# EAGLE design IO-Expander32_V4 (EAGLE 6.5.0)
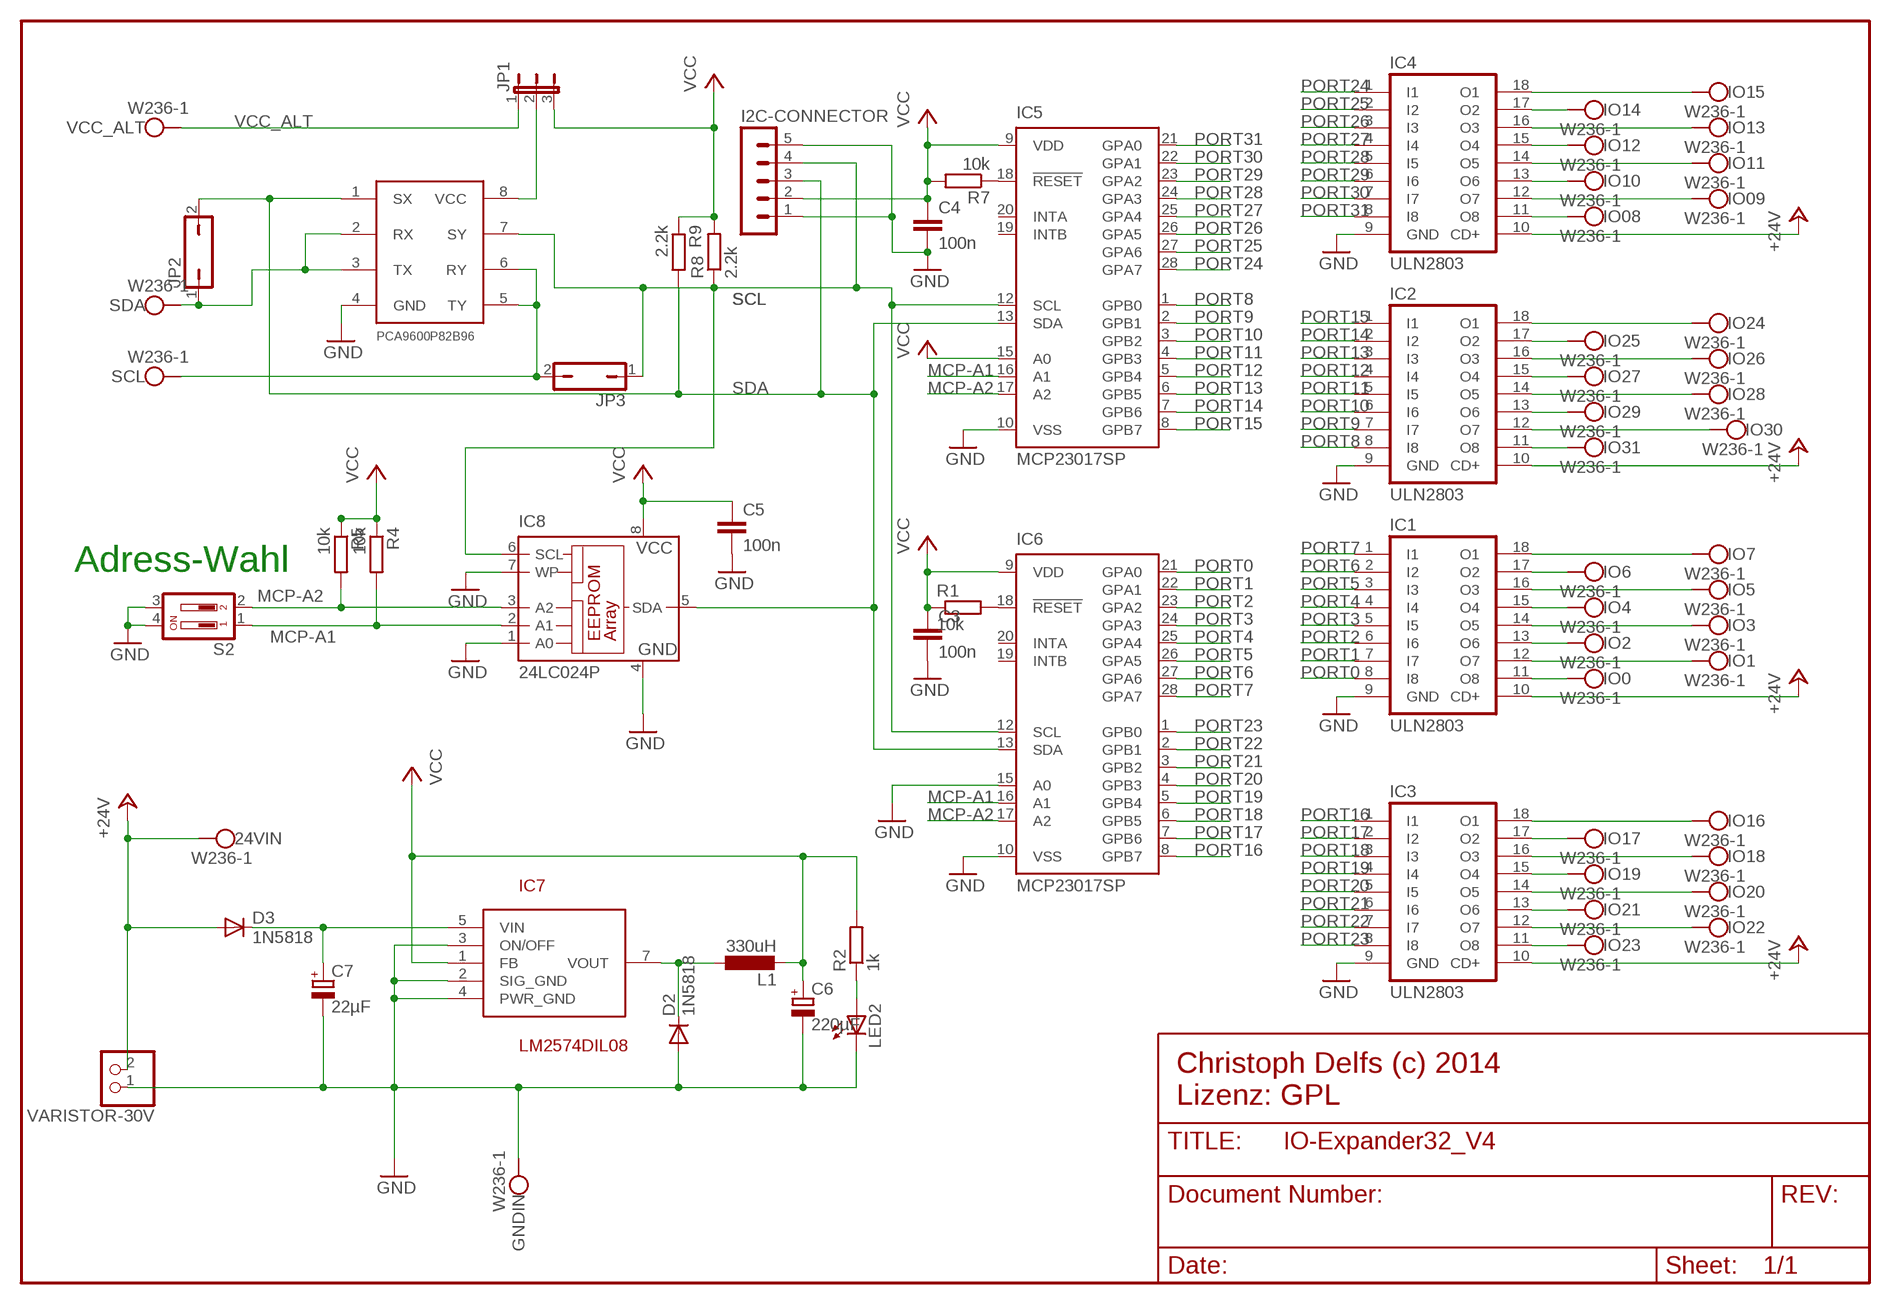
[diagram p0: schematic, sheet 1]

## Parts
24VIN  W236-1  [W236-1]
C3  100n  C-EU050-025X075  [C050-025X075]
C4  100n  C-EU050-025X075  [C050-025X075]
C5  100n  C-EU050-025X075  [C050-025X075]
C6  220µF  CPOL-EUE5-10.5  [E5-10,5]
C7  22µF  CPOL-EUE2.5-6  [E2,5-6]
D2  1N5818  1N4148  [DO35-10]
D3  1N5818  1N4148  [DO35-10]
GNDIN  W236-1  [W236-1]
I2C-CONNECTOR  MA05-1  [MA05-1]
IC1  ULN2803  ULN2803A  [DIL18]
IC2  ULN2803  ULN2803A  [DIL18]
IC3  ULN2803  ULN2803A  [DIL18]
IC4  ULN2803  ULN2803A  [DIL18]
IC5  MCP23017SP  [DIL28-3]
IC6  MCP23017SP  [DIL28-3]
IC7  LM2574DIL08  [DIL08]
IC8  24LC024P  [DIL8]
IO0  W236-1  [W236-1]
IO1  W236-1  [W236-1]
IO2  W236-1  [W236-1]
IO3  W236-1  [W236-1]
IO4  W236-1  [W236-1]
IO5  W236-1  [W236-1]
IO6  W236-1  [W236-1]
IO7  W236-1  [W236-1]
IO08  W236-1  [W236-1]
IO09  W236-1  [W236-1]
IO10  W236-1  [W236-1]
IO11  W236-1  [W236-1]
IO12  W236-1  [W236-1]
IO13  W236-1  [W236-1]
IO14  W236-1  [W236-1]
IO15  W236-1  [W236-1]
IO16  W236-1  [W236-1]
IO17  W236-1  [W236-1]
IO18  W236-1  [W236-1]
IO19  W236-1  [W236-1]
IO20  W236-1  [W236-1]
IO21  W236-1  [W236-1]
IO22  W236-1  [W236-1]
IO23  W236-1  [W236-1]
IO24  W236-1  [W236-1]
IO25  W236-1  [W236-1]
IO26  W236-1  [W236-1]
IO27  W236-1  [W236-1]
IO28  W236-1  [W236-1]
IO29  W236-1  [W236-1]
IO30  W236-1  [W236-1]
IO31  W236-1  [W236-1]
JP1  JP2E  [JP2]
JP2  JP1Q  [JP1]
JP3  JP1Q  [JP1]
L1  330uH  L-EU2200-12.7  [2200-12.7]
LED2  LED3MM  [LED3MM]
PCA9600  PCA9600  P82B96  [SOIC8]
R1  10k  R-EU_0207/2V  [0207/2V]
R2  1k  R-EU_0207/10  [0207/10]
R4  10k  R-EU_0207/7  [0207/7]
R5  10k  R-EU_0207/7  [0207/7]
R7  10k  R-EU_0207/7  [0207/7]
R8  2.2k  R-EU_0207/7  [0207/7]
R9  2.2k  R-EU_0207/7  [0207/7]
S2  DIP02YL  [DIP02YL]
SCL  W236-1  [W236-1]
SDA  W236-1  [W236-1]
VARISTOR-30V  PINHD-1X2  [1X02]
VCC_ALT  W236-1  [W236-1]

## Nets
+24V: 24VIN.1(KL1) D3.A IC1.10(CD+) IC2.10(CD+) IC3.10(CD+) IC4.10(CD+) VARISTOR-30V.2
GND: C3.2 C4.2 C5.2 C6.- C7.- D2.A GNDIN.1(KL1) I2C-CONNECTOR.1 I2C-CONNECTOR.5 IC1.9(GND) IC2.9(GND) IC3.9(GND) IC4.9(GND) IC5.10(VSS) IC6.10(VSS) IC6.15(A0) IC7.2(SIG_GND) IC7.3(ON/OFF) IC7.4(PWR_GND) IC8.1(A0) IC8.4(GND) IC8.7(WP) LED2.K(C) PCA9600.4(GND) S2.3 S2.4 VARISTOR-30V.1
IO1: IC1.18(O1) IO7.1(KL1)
IO2: IC3.16(O3) IO18.1(KL1)
IO14: IC2.16(O3) IO26.1(KL1)
IO24: IC4.18(O1) IO15.1(KL1)
MCP-A1: IC5.16(A1) IC6.16(A1) IC8.2(A1) R4.2 S2.1
MCP-A2: IC5.17(A2) IC6.17(A2) IC8.3(A2) R5.2 S2.2
N$1: LED2.A R2.1
N$2: IC6.18(!RESET) R1.2
N$4: IC4.17(O2) IO14.1(KL1)
N$5: IC4.16(O3) IO13.1(KL1)
N$7: IC4.15(O4) IO12.1(KL1)
N$8: IC4.14(O5) IO11.1(KL1)
N$9: IC4.13(O6) IO10.1(KL1)
N$10: IC4.12(O7) IO09.1(KL1)
N$11: IC5.18(!RESET) R7.1
N$12: JP1.2 PCA9600.8(VCC)
N$14: JP3.2 PCA9600.5(TY) PCA9600.6(RY) SCL.1(KL1)
N$16: JP2.1 PCA9600.2(RX) PCA9600.3(TX) SDA.1(KL1)
N$17: IC1.17(O2) IO6.1(KL1)
N$18: IC1.16(O3) IO5.1(KL1)
N$19: IC1.15(O4) IO4.1(KL1)
N$20: IC1.14(O5) IO3.1(KL1)
N$21: IC1.13(O6) IO2.1(KL1)
N$22: IC1.12(O7) IO1.1(KL1)
N$23: IC1.11(O8) IO0.1(KL1)
N$24: IC3.18(O1) IO16.1(KL1)
N$25: IC3.17(O2) IO17.1(KL1)
N$26: IC3.15(O4) IO19.1(KL1)
N$27: IC3.14(O5) IO20.1(KL1)
N$28: IC3.13(O6) IO21.1(KL1)
N$29: IC3.12(O7) IO22.1(KL1)
N$30: IC3.11(O8) IO23.1(KL1)
N$43: C7.+ D3.C IC7.5(VIN)
N$50: D2.C IC7.7(VOUT) L1.1
N$56: IC4.11(O8) IO08.1(KL1)
N$65: IC2.18(O1) IO24.1(KL1)
N$66: IC2.17(O2) IO25.1(KL1)
N$68: IC2.15(O4) IO27.1(KL1)
N$69: IC2.14(O5) IO28.1(KL1)
N$70: IC2.13(O6) IO29.1(KL1)
N$71: IC2.12(O7) IO30.1(KL1)
N$72: IC2.11(O8) IO31.1(KL1)
PORT0: IC1.8(I8) IC6.21(GPA0)
PORT1: IC1.7(I7) IC6.22(GPA1)
PORT2: IC1.6(I6) IC6.23(GPA2)
PORT3: IC1.5(I5) IC6.24(GPA3)
PORT4: IC1.4(I4) IC6.25(GPA4)
PORT5: IC1.3(I3) IC6.26(GPA5)
PORT6: IC1.2(I2) IC6.27(GPA6)
PORT7: IC1.1(I1) IC6.28(GPA7)
PORT8: IC2.8(I8) IC5.1(GPB0)
PORT9: IC2.7(I7) IC5.2(GPB1)
PORT10: IC2.6(I6) IC5.3(GPB2)
PORT11: IC2.5(I5) IC5.4(GPB3)
PORT12: IC2.4(I4) IC5.5(GPB4)
PORT13: IC2.3(I3) IC5.6(GPB5)
PORT14: IC2.2(I2) IC5.7(GPB6)
PORT15: IC2.1(I1) IC5.8(GPB7)
PORT16: IC3.1(I1) IC6.8(GPB7)
PORT17: IC3.2(I2) IC6.7(GPB6)
PORT18: IC3.3(I3) IC6.6(GPB5)
PORT19: IC3.4(I4) IC6.5(GPB4)
PORT20: IC3.5(I5) IC6.4(GPB3)
PORT21: IC3.6(I6) IC6.3(GPB2)
PORT22: IC3.7(I7) IC6.2(GPB1)
PORT23: IC3.8(I8) IC6.1(GPB0)
PORT24: IC4.1(I1) IC5.28(GPA7)
PORT25: IC4.2(I2) IC5.27(GPA6)
PORT26: IC4.3(I3) IC5.26(GPA5)
PORT27: IC4.4(I4) IC5.25(GPA4)
PORT28: IC4.5(I5) IC5.24(GPA3)
PORT29: IC4.6(I6) IC5.23(GPA2)
PORT30: IC4.7(I7) IC5.22(GPA1)
PORT31: IC4.8(I8) IC5.21(GPA0)
SCL: I2C-CONNECTOR.4 IC5.12(SCL) IC6.12(SCL) IC8.6(SCL) JP3.1 PCA9600.7(SY) R8.1
SDA: I2C-CONNECTOR.3 IC5.13(SDA) IC6.13(SDA) IC8.5(SDA) JP2.2 PCA9600.1(SX) R9.2
VCC: C3.1 C4.1 C5.1 C6.+ I2C-CONNECTOR.2 IC5.9(VDD) IC5.15(A0) IC6.9(VDD) IC7.1(FB) IC8.8(VCC) JP1.3 L1.2 R1.1 R2.2 R4.1 R5.1 R7.2 R8.2 R9.1
VCC_ALT: JP1.1 VCC_ALT.1(KL1)
Unconnected: 24VIN.2(KL2) GNDIN.2(KL2) IC5.19(INTB) IC5.20(INTA) IC6.19(INTB) IC6.20(INTA) IO0.2(KL2) IO1.2(KL2) IO2.2(KL2) IO3.2(KL2) IO4.2(KL2) IO5.2(KL2) IO6.2(KL2) IO7.2(KL2) IO08.2(KL2) IO09.2(KL2) IO10.2(KL2) IO11.2(KL2) IO12.2(KL2) IO13.2(KL2) IO14.2(KL2) IO15.2(KL2) IO16.2(KL2) IO17.2(KL2) IO18.2(KL2) IO19.2(KL2) IO20.2(KL2) IO21.2(KL2) IO22.2(KL2) IO23.2(KL2) IO24.2(KL2) IO25.2(KL2) IO26.2(KL2) IO27.2(KL2) IO28.2(KL2) IO29.2(KL2) IO30.2(KL2) IO31.2(KL2) SCL.2(KL2) SDA.2(KL2) VCC_ALT.2(KL2)

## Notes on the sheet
- Adress-Wahl
- Christoph Delfs (c) 2014
  Lizenz: GPL

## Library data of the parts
24VIN GNDIN IO0 IO1-IO7 IO08 IO09 IO10-IO31 SCL SDA VCC_ALT = con-wago-508:W236-1: WAGO SREW CLAMP
C3-C5 = rcl:C-EU: CAPACITOR, European symbol
C6 C7 = rcl:CPOL-EU: POLARIZED CAPACITOR, European symbol
D2 D3 = diode:1N4148: DIODE
I2C-CONNECTOR = con-lstb:MA05-1: PIN HEADER; OC_FARNELL: unknown; OC_NEWARK: unknown
IC1-IC4 = uln-udn:ULN2803A: DRIVER ARRAY
IC5 IC6 = microchip:MCP23017: http://ww1.microchip.com/downloads/en/DeviceDoc/21952a.pdf Source: http://ww1.microchip.com/downloads/en/DeviceDoc/21952a.pdf; MF: MICROCHIP; MPN: MCP23017-E/SP; OC_FARNELL: 1332088; OC_NEWARK: 31K2959
IC7 = hausbus-bauteile:LM2574
IC8 = microchip:24*: Serial EEPROM I2C; MPN: 24LC024-I/P; OC_FARNELL: 1331317; OC_NEWARK: 35M0731
JP1 = jumper:JP2E: JUMPER
JP2 JP3 = jumper:JP1Q: JUMPER
L1 = rcl:L-EU: INDUCTOR, European symbol
LED2 = led:LED: LED
PCA9600 = P82B96:P82B96: P82B96 - I2C buffer
R1 R2 R4 R5 R7-R9 = rcl:R-EU_: RESISTOR, European symbol
S2 = switch-dil:DIP02YL: DIL/CODE SWITCH; OC_FARNELL: unknown; OC_NEWARK: unknown
VARISTOR-30V = pinhead:PINHD-1X2: PIN HEADER

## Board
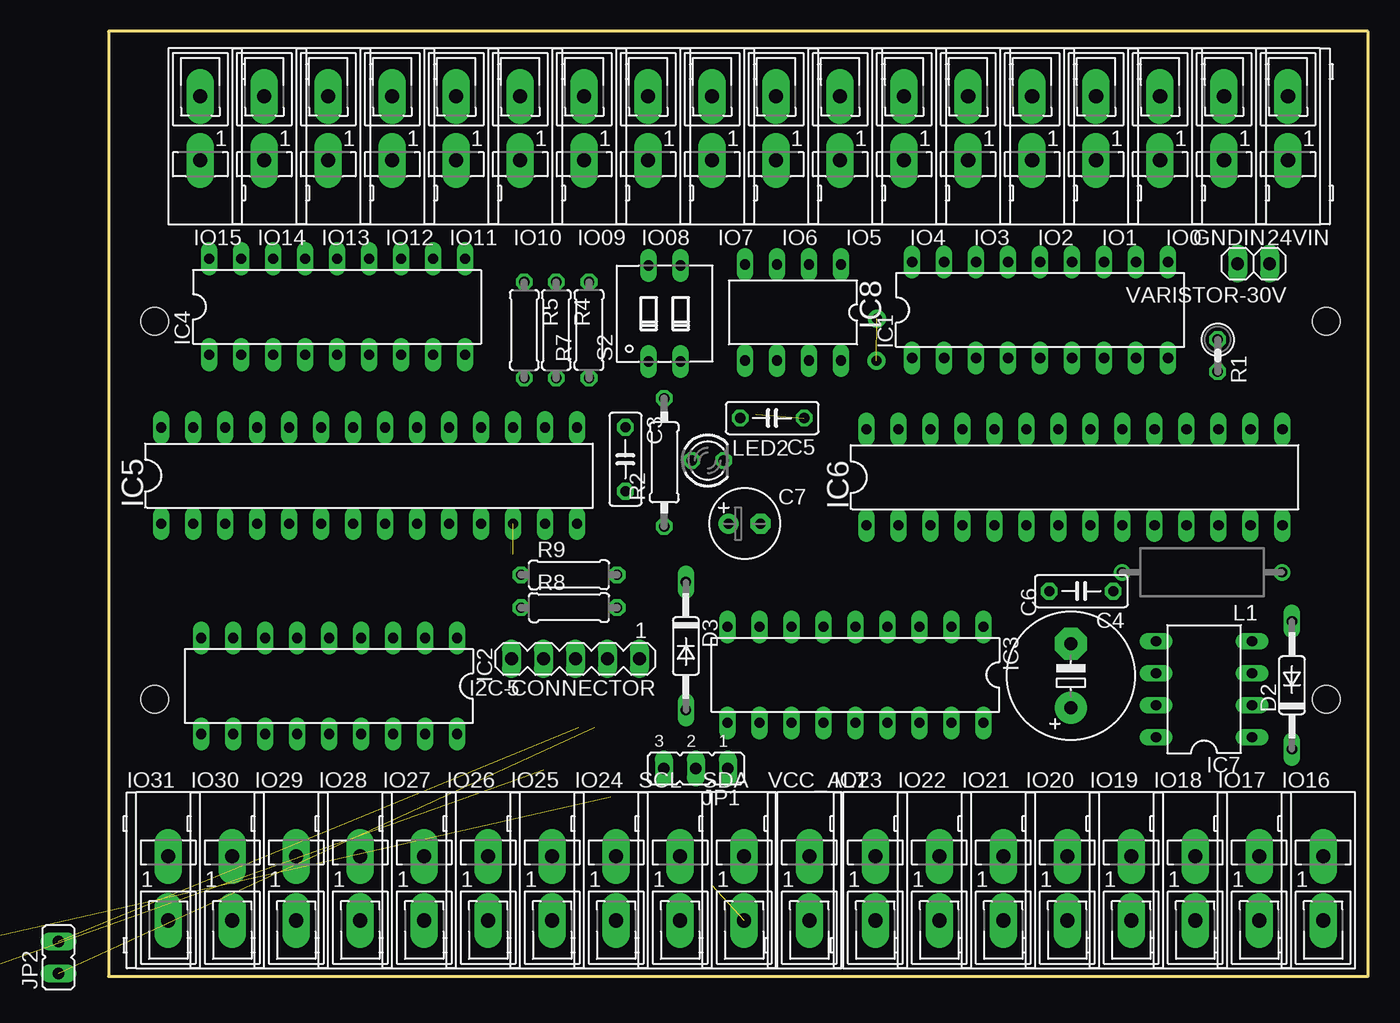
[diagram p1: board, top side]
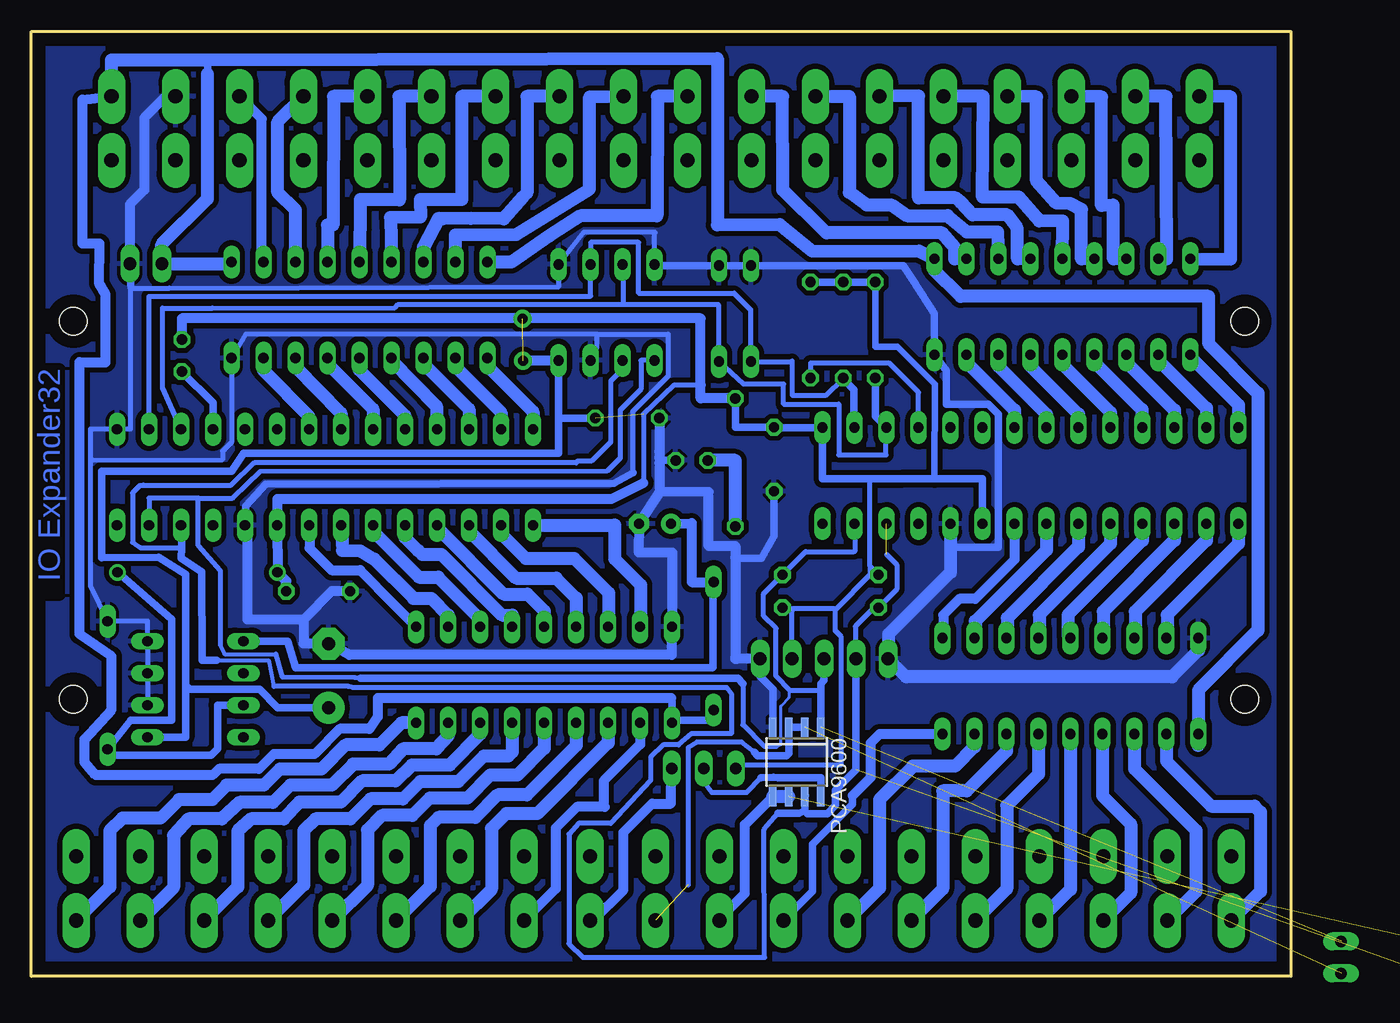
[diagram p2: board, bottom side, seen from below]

Size 100 x 75 mm. Coordinates in mm from the lower left corner, seen from the top.
Outline: 100,0 100,75 0,75 0,0 100,0
Copper layers (1*16): Top 0.035mm / dielectric 1.5mm / Bottom 0.035mm
Design rules "default": minimum track width 10mil, minimum drill 24mil, track to track 8mil, track to pad 8mil, pad to pad 8mil, via to via 8mil, smd to smd 8mil, copper to edge 40mil, drill to drill 8mil, minimum pad ring 10mil, minimum via ring 8mil, stop-mask expansion 4mil, vias tented up to drill 0mil, thermal gap 10mil
Holes 2.2 mm at 3.67,22 3.67,52 96.67,22 96.67,52

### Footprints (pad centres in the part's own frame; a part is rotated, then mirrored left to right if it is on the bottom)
W236-1 = drill 1.118 pad 2.184 long: 1 0,-2.54; 2 0,2.54
C050-025X075 = drill 0.813 octagon: 1 -2.54,0; 2 2.54,0
E5-10,5 = drill 1.016 pad 2.54: + -2.54,0 | drill 1.016 pad 2.54 octagon: - 2.54,0
E2,5-6 = drill 0.813 pad 1.6: + -1.27,0 | drill 0.813 pad 1.6 octagon: - 1.27,0
DO35-10 = drill 0.813 long: A 5.08,0; C -5.08,0
MA05-1 = drill 1.016 long: 1 -5.08,0; 2 -2.54,0; 3 0,0; 4 2.54,0; 5 5.08,0
DIL18 = drill 0.813 long: 1 -10.16,-3.81; 2 -7.62,-3.81; 3 -5.08,-3.81; 4 -2.54,-3.81; 5 0,-3.81; 6 2.54,-3.81; 7 5.08,-3.81; 8 7.62,-3.81; 9 10.16,-3.81; 10 10.16,3.81; 11 7.62,3.81; 12 5.08,3.81; 13 2.54,3.81; 14 0,3.81; 15 -2.54,3.81; 16 -5.08,3.81; 17 -7.62,3.81; 18 -10.16,3.81
DIL28-3 = drill 0.813 long: 1 -16.51,-3.81; 2 -13.97,-3.81; 3 -11.43,-3.81; 4 -8.89,-3.81; 5 -6.35,-3.81; 6 -3.81,-3.81; 7 -1.27,-3.81; 8 1.27,-3.81; 9 3.81,-3.81; 10 6.35,-3.81; 11 8.89,-3.81; 12 11.43,-3.81; 13 13.97,-3.81; 14 16.51,-3.81; 15 16.51,3.81; 16 13.97,3.81; 17 11.43,3.81; 18 8.89,3.81; 19 6.35,3.81; 20 3.81,3.81; 21 1.27,3.81; 22 -1.27,3.81; 23 -3.81,3.81; 24 -6.35,3.81; 25 -8.89,3.81; 26 -11.43,3.81; 27 -13.97,3.81; 28 -16.51,3.81
DIL08 = drill 0.813 long: 1 -3.81,-3.81; 2 -1.27,-3.81; 3 1.27,-3.81; 4 3.81,-3.81; 5 3.81,3.81; 6 1.27,3.81; 7 -1.27,3.81; 8 -3.81,3.81
DIL8 = drill 0.813 long: 1 -3.81,-3.81; 2 -1.27,-3.81; 3 1.27,-3.81; 4 3.81,-3.81; 5 3.81,3.81; 6 1.27,3.81; 7 -1.27,3.81; 8 -3.81,3.81
JP2 = drill 0.914 long: 1 -2.54,0; 2 0,0; 3 2.54,0
JP1 = drill 0.914 long: 1 0,-1.27; 2 0,1.27
2200-12.7 = drill 0.8 pad 1.27: 1 -6.35,0; 2 6.35,0
LED3MM = drill 0.813 octagon: A -1.27,0; K 1.27,0
SOIC8 = smd 0.6 x 1.5: 1 -1.905,-2.75; 2 -0.635,-2.75; 3 0.635,-2.75; 4 1.905,-2.75; 5 1.905,2.75; 6 0.635,2.75; 7 -0.635,2.75; 8 -1.905,2.75
0207/2V = drill 0.813 octagon: 1 -1.27,0; 2 1.27,0
0207/10 = drill 0.813 octagon: 1 -5.08,0; 2 5.08,0
0207/7 = drill 0.813 octagon: 1 -3.81,0; 2 3.81,0
DIP02YL = drill 0.813 long: 1 -1.27,-3.81; 2 1.27,-3.81; 3 1.27,3.81; 4 -1.27,3.81
1X02 = drill 1.016 long: 1 -1.27,0; 2 1.27,0

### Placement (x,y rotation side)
24VIN  93.65,67.31 180 top
C3  41.04,41.05 270 top
C4  77.24,30.58 180 top
C5  52.69,44.32 180 top
C6  76.41,23.88 90 top
C7  50.5,35.94 0 top
D2  93.97,23.11 90 top
D3  45.83,26.23 270 top
GNDIN  88.57,67.31 180 top
I2C-CONNECTOR  37.07,25.21 180 top
IC1  73.97,52.9 0 top
IC2  17.51,23.05 180 top
IC3  59.3,23.94 180 top
IC4  18.15,53.15 0 top
IC5  20.69,39.75 0 top
IC6  76.7,39.62 0 top
IC7  86.98,22.8 90 top
IC8  54.34,52.7 180 top
IO0  83.49,67.31 180 top
IO1  78.41,67.31 180 top
IO2  73.33,67.31 180 top
IO3  68.25,67.31 180 top
IO4  63.17,67.31 180 top
IO5  58.09,67.31 180 top
IO6  53.01,67.31 180 top
IO7  47.93,67.31 180 top
IO08  42.85,67.31 180 top
IO09  37.77,67.31 180 top
IO10  32.69,67.31 180 top
IO11  27.61,67.31 180 top
IO12  22.53,67.31 180 top
IO13  17.45,67.31 180 top
IO14  12.37,67.31 180 top
IO15  7.29,67.31 180 top
IO16  96.44,6.99 0 top
IO17  91.36,6.99 0 top
IO18  86.28,6.99 0 top
IO19  81.2,6.99 0 top
IO20  76.12,6.99 0 top
IO21  71.04,6.99 0 top
IO22  65.96,6.99 0 top
IO23  60.88,6.99 0 top
IO24  40.31,6.99 0 top
IO25  35.23,6.99 0 top
IO26  30.15,6.99 0 top
IO27  25.07,6.99 0 top
IO28  19.99,6.99 0 top
IO29  14.91,6.99 0 top
IO30  9.83,6.99 0 top
IO31  4.75,6.99 0 top
JP1  46.63,16.51 180 top
JP2  not placed on the board
JP3  not placed on the board
L1  86.82,32.07 180 top
LED2  47.58,40.96 0 top
PCA9600  39.23,17.02 180 bottom
R1  88.06,49.28 270 top
R2  44.12,40.8 90 top
R4  35.55,51.31 270 top
R5  33.01,51.31 270 top
R7  38.15,51.31 90 top
R8  36.56,29.27 0 top
R9  36.56,31.88 0 top
S2  44.15,52.61 0 top
SCL  45.39,6.99 0 top
SDA  50.47,6.99 0 top
VARISTOR-30V  90.92,56.58 180 top
VCC_ALT  55.65,6.99 0 top

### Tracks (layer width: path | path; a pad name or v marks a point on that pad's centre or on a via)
+24V
  Bottom 0.61: 86.03,71.63 86.03,72.75 | D3.A 45.83,20.67 46.15,20.35 48.91,20.35 IC3.10 49.14,22.04 49.2,22.1
  Bottom 0.813: 49.2,22.1 72.5,22.1 72.5,20.61 73.17,19.65 75.52,19.65 77.52,17.65 80.76,17.65 81.93,16.48 85.11,16.48 85.62,15.97 94.89,15.97 95.78,17.02 95.78,18.83 93.65,21.18 93.65,25.4 96.19,27.18 96.19,48.77 94.13,48.74 94.13,54.13 94.63,55.02 94.6,58.17 95.94,58.17 95.94,69.6 24VIN.1
  Bottom 1.016: 24VIN.1 93.65,72.74 86.03,72.75 86,72.75 45.55,72.87 45.55,59.66 40.6,59.69 38.02,57.59 29.52,57.56 IC4.10 28.37,56.9 28.37,56.13 26.21,53.98 6.56,53.98 6.56,50.26 2.62,46.29 2.62,27.46 7.35,22.7 IC2.10 7.38,18.32 | 86.03,71.63 86.03,61.72 89.65,58.1 VARISTOR-30V.2 84.25,56.58 IC1.10
GND
  Bottom 0.406: IC8.1 56.19,59.05 50.47,59.05 50.53,58.99 IC8.4 | 58.09,56.52 IC8.1 | 95.3,40.99 84.82,41.02 84.82,41.69 84.12,42.39 IC1.9 82.98,50.99 55.11,50.99 | 55.11,50.99 49.45,50.99 49.45,47.62 52.25,44.86 52.25,39.97 | IC8.7 55.11,49.97 55.11,50.99 | IC8.1 58.15,54.74 89.05,54.64 92.19,54.64 92.13,54.86 92.13,43.43 IC6.15 95.3,43.43 95.3,40.99 | 95.3,40.83 95.3,40.99 | 95.3,40.83 95.24,41.05 95.3,40.99 | 95.3,40.83 95.3,30.99 D2.A 90.79,28.19 IC7.4 IC7.3 IC7.2 90.86,21.53 90.86,21.59
  Bottom 0.61: 92.13,54.86 VARISTOR-30V.1 | PCA9600.4 41.14,22.8 42.15,23.84 I2C-CONNECTOR.1 | 52.25,39.97 53.74,39.15 81.39,39.05 83.01,37.31 IC6.10 | 26.85,31.91 27.04,32.1 | IC8.4 50.53,56.42 S2.3 S2.4 30.75,56.42 29.93,55.15 28.31,52.61 IC4.9 27.36,48.07 27.36,45.43 24.02,45.43 23.23,44.64 23.23,34.07 27.04,34.07 IC5.10 | C3.2 41.04,34.92 42.06,33.18 44.06,33.18 44.12,33.24 | 50.15,41.18 | LED2.K 49.93,40.96 50.15,40.73
  Bottom 0.813: GNDIN.1 89.33,69.85 91.05,68.14 91.05,62.42 92.19,61.28 VARISTOR-30V.1 | C5.2 50.15,41.66 50.15,41.18 50.15,40.73 50.15,38.45 | 50.15,38.45 50.15,38.39 C7.- 51.8,33.66 49.14,33.66 IC3.9 49.17,25.75 49.17,25.53 74.76,25.53 C6.- 78.41,26.42 78.41,28.32 | 50.15,38.45 46.25,38.45 46.25,34.16 44.12,34.16 44.12,33.24 44.12,25.3 | 44.12,25.3 44.12,25.21 | 78.41,28.32 82.86,28.32 82.86,35.62 IC6.10 | I2C-CONNECTOR.1 44.02,25.21 44.12,25.3 | C4.2 76.16,30.57 78.41,28.32
  Bottom 1.016: IC2.9 7.35,25.88 9.45,23.78 30.56,23.78 I2C-CONNECTOR.5 31.96,25.24 31.96,27.18 27.04,32.1 IC5.10
  pour Bottom (isolate 0.406): -0.33,74.93 100,74.93 100,0 -0.33,0
IO1
  Bottom 1.016: IO7.1 50.31,69.85 50.34,60.36 56.41,60.36 58.88,58.77 61.9,56.71 IC1.18
IO2
  Bottom 1.016: IC3.16 64.38,19.24 66.79,16.76 69.81,16.76 71.11,15.53 73.74,15.53 75.42,13.84 78.73,13.84 79.97,12.51 82.57,12.51 83.62,11.56 83.62,7.11 IO18.1
IO14
  Bottom 1.016: IC2.16 22.59,17.88 25.74,14.73 27.64,14.73 27.64,6.95 IO26.1
IO24
  Bottom 1.016: IC4.18 4.78,56.93 4.78,69.82 IO15.1
MCP-A1
  Bottom 0.406: 39.61,48.83 39.61,48.74 | 39.61,48.74 39.61,46.13 36.91,46.13 R4.2 | IC6.16 90.67,53.98 87.36,53.98 55.61,54.01 IC8.2 55.61,58.26 51.8,58.26 51.8,54.23 44.22,54.23 42.91,52.93 42.91,48.83 S2.1 39.68,48.8 39.61,48.74
  Bottom 0.61: R4.2 35.55,47.43 34.69,46.58 34.69,43.59 IC5.16
MCP-A2
  Bottom 0.406: 53.04,53.34 70.89,53.34 71.14,53.09 85.62,53.05 89.59,53.05 89.59,46.74 IC6.17 | 53.04,53.34 45.52,53.34 45.42,53.24 S2.2 43.48,47.02 40.28,47.02 40.28,45.43 35.9,45.43 35.9,41.4 32.15,41.4 IC5.17 | IC8.3 53.04,56.52 53.04,53.34
  Bottom 0.61: R5.2 33.01,44.45 IC5.17
N$1
  Bottom 1.016: R2.1 44.12,40.96 LED2.A
N$2
  Bottom 0.61: IC6.18 85.59,45.53 R1.2
N$4
  Bottom 1.016: IC4.17 9.86,56.96 9.93,69.85 IO14.1
N$5
  Bottom 1.016: IC4.16 14.08,56.93 14.12,61.21 15.04,61.18 15.04,69.82 IO13.1
N$7
  Bottom 1.016: IC4.15 16.62,56.93 16.62,60.87 17.55,61.34 18.62,61.37 20.21,63.15 20.21,69.82 IO12.1
N$8
  Bottom 1.016: IC4.14 18.12,59.94 19.99,59.98 21.61,61.85 24.5,61.85 24.44,69.85 IO11.1
N$9
  Bottom 1.016: IC4.13 21.71,56.96 21.74,59.37 22.53,60.45 25.29,60.45 26.21,61.44 26.63,61.78 29.58,61.78 29.58,69.88 IO10.1
N$10
  Bottom 1.016: IO09.1 35.07,69.85 35.07,62.23 33.71,61.25 31.74,61.25 30.5,60.39 27.26,60.39 25.74,59.09 23.29,59.09 IC4.12
N$11
  Bottom 0.406: R7.1 38.15,48.7 31.93,48.7 29.58,46.35 IC5.18
N$12
  Bottom 0.406: JP1.2 46.66,15.49 45.99,14.61 43.2,14.61 42.09,15.78
  Bottom 0.61: 42.09,15.78 41.07,15.81 40.72,15.78 37.33,15.78 PCA9600.8
N$14  (1 unrouted)
  Bottom 0.813: SCL.1 45.39,4.57 43.36,6.6 43.36,12.05 PCA9600.5
  Bottom 1.016: PCA9600.6 PCA9600.5
N$16  (2 unrouted)
  Bottom 0.406: 42.6,17.78 43.61,18.61 47.17,18.61 47.87,18.16 47.87,7.27
  Bottom 0.61: PCA9600.2 PCA9600.3 39.87,17.72 40.06,17.53 42.34,17.53 42.6,17.78
N$17
  Bottom 1.016: IC1.17 66.34,58.86 61.49,58.9 55.71,62.48 55.68,69.82 IO6.1
N$18
  Bottom 1.016: IO5.1 60.66,69.85 60.66,62.2 60.98,61.88 62.5,60.13 65.11,60.17 67.36,60.13 67.68,60.17 68.89,57.91 IC1.16
N$19
  Bottom 1.016: IO4.1 65.84,69.85 65.84,61.66 69.14,61.66 69.11,60.26 71.49,60.23 IC1.15
N$20
  Bottom 1.016: IO3.1 70.82,69.85 70.79,61.63 73.9,61.66 IC1.14
N$21
  Bottom 1.016: IO2.1 76.03,69.85 76.06,59.63 76.5,59.63 IC1.13
N$22
  Bottom 1.016: IC1.12 79.05,60.83 80.44,62.23 80.44,67.82 IO1.1
N$23
  Bottom 0.813: IC1.11 81.74,56.74 81.74,60.93 81.71,68.07 IO0.1
N$24
  Bottom 1.016: IC3.18 70.63,20.13 72.38,18.38 75.04,18.38 76.98,16.45 80.28,16.45 81.55,15.18 84.51,15.18 85.65,14.03 88.28,14.03 89.75,12.57 92.79,12.57 93.78,11.59 93.78,7.11 IO16.1
N$25
  Bottom 1.016: IC3.17 66.92,19.11 67.87,18.07 70.5,18.07 71.61,16.86 74.47,16.86 76.16,15.18 79.46,15.18 80.82,13.81 83.49,13.81 84.89,12.51 87.52,12.51 88.73,11.21 88.73,7.08 IO17.1
N$26
  Bottom 1.016: IC3.15 61.84,17.81 62.15,17.49 64.09,17.49 66.12,15.46 69.14,15.46 70.5,14.1 73.08,14.1 74.66,12.51 77.46,12.51 78.38,11.59 78.38,7.27 IO19.1
N$27
  Bottom 1.016: IC3.14 59.3,18.1 61.42,15.97 63.58,15.97 65.39,14.16 68.38,14.16 69.74,12.79 72.16,12.79 73.33,11.62 73.33,7.24 IO20.1
N$28
  Bottom 1.016: IC3.13 56.76,18.32 60.66,14.41 62.98,14.41 64.76,12.64 67.68,12.64 68.34,11.97 68.34,7.14 IO21.1
N$29
  Bottom 1.016: IC3.12 54.22,18.54 59.84,12.92 62.31,12.92 63.49,11.75 63.49,6.92 IO22.1
N$30
  Bottom 0.813: IC3.11 51.68,18.41 54.57,15.53 54.57,13.56 54.47,13.46 56.69,13.46 58.38,11.78 58.38,6.95 IO23.1
N$43
  Bottom 0.61: IC7.5 79.68,26.61 79.05,24.51 45.93,24.51 45.9,24.54 45.9,31.24 D3.C
  Bottom 0.813: C7.+ 47.58,35.97 47.58,31.3 D3.C
N$50
  Bottom 0.61: L1.1 88.86,28.35 88.86,20.32 92.13,20.32 D2.C 93.97,17.56 85.74,17.56 85.24,18.07 85.24,21.53 IC7.7
N$56
  Bottom 1.016: IC4.11 26.69,56.96 26.69,57.85 27.71,59.02 36.88,59.02 40.34,62.42 40.37,69.85 IO08.1
N$65
  Bottom 0.61: 34.82,14.35 34.82,13.65 37.99,10.48 37.99,6.76 IO24.1
  Bottom 0.813: IC2.18 32.66,19.24 33.39,18.51 33.39,15.78 34.82,14.35
N$66
  Bottom 1.016: IC2.17 25.13,18.22 26.66,16.7 30.02,16.7 32.66,14.06 32.66,7.02 IO25.1
N$68
  Bottom 1.016: IC2.15 20.05,16.07 22.56,13.56 22.56,6.95 IO27.1
N$69
  Bottom 1.016: IC2.14 17.51,6.92 IO28.1
N$70
  Bottom 1.016: IC2.13 14.97,14.35 12.72,12.1 12.72,6.64 IO29.1
N$71
  Bottom 1.016: IC2.12 12.43,16.48 7.54,11.59 7.54,6.73 IO30.1
N$72
  Bottom 1.016: IC2.11 9.89,17.08 6.34,13.53 2.91,13.53 2.43,13.05 2.43,6.76 IO31.1
PORT0
  Bottom 1.016: IC1.8 81.59,48.13 77.97,44.45 IC6.21
PORT1
  Bottom 1.016: IC1.7 79.05,48.39 75.42,44.7 IC6.22
PORT2
  Bottom 1.016: IC1.6 76.5,48.64 72.89,45.02 IC6.23
PORT3
  Bottom 1.016: IC1.5 73.97,48.13 70.34,44.51 IC6.24
PORT4
  Bottom 1.016: IC1.4 71.42,48.9 67.84,45.28 67.84,43.47 IC6.25
PORT5
  Bottom 1.016: IC1.3 68.89,48.64 65.27,45.02 IC6.26
PORT6
  Bottom 1.016: IC1.2 66.34,48.39 62.73,44.77 IC6.27
PORT7
  Bottom 1.016: IC1.1 63.81,48.45 60.19,44.83 IC6.28
PORT8
  Bottom 1.016: IC5.1 4.18,34.35 9.83,28.7 9.83,26.92 IC2.8
PORT9
  Bottom 1.016: IC5.2 6.72,34.61 12.37,28.96 12.37,26.92 IC2.7
PORT10
  Bottom 1.016: IC5.3 9.26,34.61 14.91,28.96 14.91,26.92 IC2.6
PORT11
  Bottom 1.016: IC5.4 11.8,34.61 17.7,28.7 17.7,27.05 IC2.5
PORT12
  Bottom 1.016: IC5.5 14.34,34.35 19.99,28.7 19.99,26.92 IC2.4
PORT13
  Bottom 1.016: IC5.6 16.88,34.1 22.53,28.45 22.53,26.92 IC2.3
PORT14
  Bottom 1.016: IC5.7 19.42,33.85 25.07,28.19 25.07,26.92 IC2.2
PORT15
  Bottom 0.813: IC5.8 21.96,33.08 25.07,29.97 26.34,29.97 27.61,28.7 27.61,26.92 IC2.1
PORT16
  Bottom 0.813: IC3.1 71.27,29.56 73.9,32.26 76.19,32.26 77.93,34 IC6.8
PORT17
  Bottom 1.016: IC6.7 75.3,33.81 73.9,33.78 72.79,33.12 69.68,30 68.25,30 66.92,28.67 IC3.2
PORT18
  Bottom 1.016: IC6.6 72.89,35.34 69.23,31.69 67.71,31.69 64.38,28.35 IC3.3
PORT19
  Bottom 1.016: IC6.5 70.34,34.83 69.33,33.81 69.3,33.81 68.98,33.5 67.46,33.5 62.63,28.67 61.84,28.67 IC3.4
PORT20
  Bottom 1.016: IC6.4 67.81,35.66 62.5,30.35 60.63,30.35 59.3,29.02 IC3.5
PORT21
  Bottom 1.016: IC6.3 65.27,35.37 61.52,31.62 58.34,31.62 56.76,30.04 IC3.6
PORT22
  Bottom 1.016: IC6.2 62.73,35.15 60.76,33.18 56.91,33.18 54.19,30.45 54.19,27.78 IC3.7
PORT23
  Bottom 1.016: IC6.1 53.74,35.81 53.71,35.85 53.71,33.15 51.65,31.08 51.65,27.78 IC3.8
PORT24
  Bottom 1.016: IC4.1 7.99,49.18 4.18,45.37 IC5.28
PORT25
  Bottom 1.016: IC4.2 10.53,48.93 6.72,45.12 IC5.27
PORT26
  Bottom 1.016: IC4.3 13.07,48.77 9.26,44.96 IC5.26
PORT27
  Bottom 1.016: IC4.4 15.61,48.77 11.83,44.99 11.83,43.59 IC5.25
PORT28
  Bottom 1.016: IC4.5 18.15,48.58 14.34,44.77 IC5.24
PORT29
  Bottom 1.016: IC4.6 20.69,48.45 16.88,44.64 IC5.23
PORT30
  Bottom 1.016: IC4.7 23.23,48.42 19.42,44.61 IC5.22
PORT31
  Bottom 1.016: IC4.8 25.77,48.77 21.96,44.96 IC5.21
SCL  (2 unrouted)
  Bottom 0.305: 85.3,25.08 81.17,25.08 80.76,23.02
  Bottom 0.406: 80.76,23.02 74.85,23.02 74.47,22.92 44.79,22.92 44.44,22.45 44.44,19.27 47.58,19.27 48.63,18.38 49.84,18.38 50.85,17.4 50.85,15.59 54.03,12.16 56.57,12.16 57.33,11.3 57.33,2.6 56.22,1.52 41.8,1.52 41.83,11.68 40.72,12.95 | 38.37,12.92 38.59,13.14 | 32.12,33.5 31.29,32.67 31.29,30.73 R8.1 33.1,29.27 34.59,27.78 34.59,26.35 34.53,26.29 | 91.08,38.96 84.19,38.96 82.31,40.77 56.76,40.77 56.63,40.89 55.55,40.89 54.03,42.42 54.03,47.24 53.07,48.2 IC8.6 | 91.08,38.96 91.11,38.99 | 91.08,38.96 91.4,38.96 91.97,38.39 91.97,34.45 91.36,34.04 88.09,34.04
  Bottom 0.61: 34.53,26.29 I2C-CONNECTOR.4 34.53,16.41 36.15,14.8 36.15,13.59 36.82,12.92 38.37,12.92 | IC6.12 88.09,34.04 88.13,33.21 86.48,32.13 86.44,25.08 85.3,25.08 | 38.53,14.33 PCA9600.7 38.59,13.14 39.07,12.95 40.72,12.95
SDA  (1 unrouted)
  Bottom 0.254: 40.88,23.81 40.85,23.81 39.87,22.83 39.87,22.13 40.5,21.46 40.5,18.45 40.82,18.29
  Bottom 0.305: 80.6,25.59 84.67,25.59 85.01,26.29
  Bottom 0.406: 80.6,25.59 80.09,23.75 74.31,23.72 73.87,23.69 | I2C-CONNECTOR.3 37.07,23.56 | 85.01,26.29 85.01,32.19 86.76,34.2 86.76,37.97 | IC8.5 51.61,48.9 51.61,46.61 53.26,44.96 53.26,41.15 54.31,40.1 81.84,40.07 84,38.01 84.03,37.97 86.76,37.97 | 37.33,22.77 37.36,22.73 39.8,22.73 40.88,23.81 40.88,27.62 41.87,28.61 41.87,30.39 R9.2 38.53,33.72 34.69,33.72 34.59,33.81 34.59,35.88 IC5.13 | 86.76,37.97 90.67,37.97 IC6.13 | 43.52,23.24 43.52,19.97 41.83,18.29 40.82,18.29
  Bottom 0.61: I2C-CONNECTOR.3 37.07,23.5 37.33,23.24 37.33,22.77 PCA9600.1 | 43.52,23.24 43.9,23.69 73.87,23.69
VCC  (via drill 0.8 pad 1.42)  (2 unrouted)
  Bottom 0.406: 51.42,39.18 51.42,44.64 48.98,46.93 46.88,46.93 | 33.42,32.54 33.42,39.5 | 33.42,32.54 R9.1 | 36.18,29.11 36.18,27.43 35.74,26.99 35.74,16.76 43.83,16.76 JP1.3 | 36.18,29.11 36.25,29.18 39.8,29.18 | 39.8,29.18 40.28,29.18 R8.2 | 33.42,32.54 33.42,31.88 36.18,29.11 | I2C-CONNECTOR.2 39.61,28.99 39.8,29.18
  Bottom 0.508: 28.31,39.48 28.28,47.02 31.23,49.97 33.01,49.97 R5.1
  Bottom 0.61: IC7.1 87.78,18.99 87.78,23.11 | 87.78,23.11 87.75,31.91 89.9,33.27 94.44,33.24 94.44,40.1 84.12,40.1 83.14,41.53 58.15,41.53 58.15,44.32 | 58.15,44.32 58.15,48.86 IC8.8 | C5.1 58.15,44.32 | IC5.9 24.5,39.5 28.31,39.48 30.94,39.5 33.42,39.5 37.2,39.5 IC5.15 40.44,43.56 C3.1 44.12,43.59 R2.2 | R5.1 R4.1 R7.2 | C6.+ 80.44,21.34 81.9,22.8 87.43,22.8 87.78,23.11
  Bottom 0.813: 51.42,39.18 53.96,37.91 80.47,37.91 80.47,35.81 IC6.9 L1.2 79.78,31.37 C4.1 | 58.15,48.86 v60.98,48.86 | R1.1 88.06,52.23 46.88,52.23 46.88,46.93 46.88,45.88 R2.2
  other vias: 61.01,52.2
VCC_ALT
  Bottom 0.813: VCC_ALT.1 55.42,4.45 53.01,6.86 53.01,11.43 50.72,13.72 49.23,13.72 JP1.1

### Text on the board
Bottom: IO Expander32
